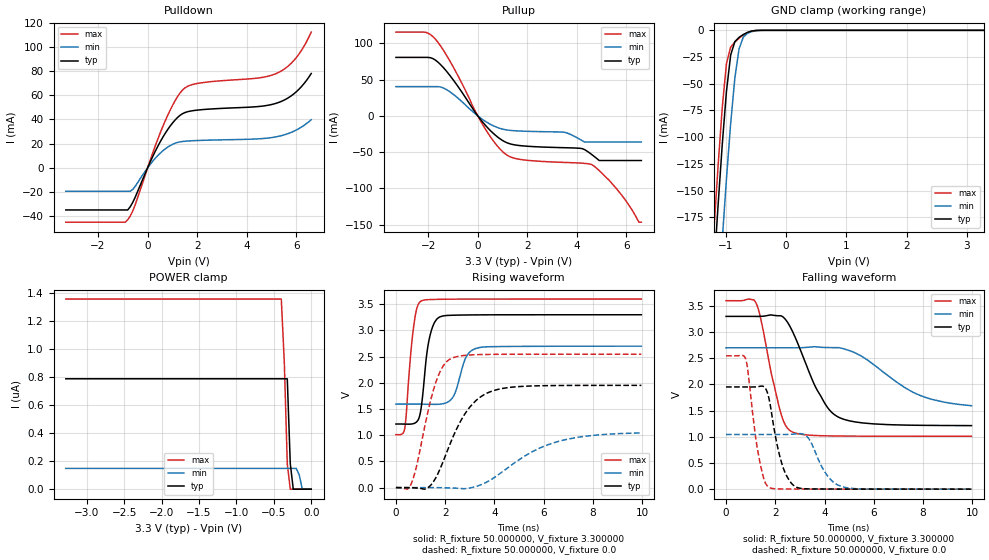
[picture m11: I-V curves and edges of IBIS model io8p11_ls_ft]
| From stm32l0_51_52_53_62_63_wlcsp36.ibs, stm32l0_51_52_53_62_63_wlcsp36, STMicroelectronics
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|   Model io8p11_ls_ft
[Model]  io8p11_ls_ft
Model_type I/O
Polarity   Non-Inverting
Enable   Active-Low
Vinl =   0.990000V
Vinh =   2.310000V
Vmeas =  1.650000V
Cref =   50.000000pF
Rref =   100.000000M
Vref =   0.0V
C_comp   4.606100pF   4.563500pF   4.706200pF
[Temperature Range]   25.000000   0.125000k   -40.000000
[Pullup Reference]   3.300000V   2.700000V   3.600000V
[Pulldown Reference]   0.0V   0.0V   0.0V
[POWER Clamp Reference]   3.300000V   2.700000V   3.600000V
[GND Clamp Reference]   0.0V   0.0V   0.0V
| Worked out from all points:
|   slope of the pulldown table from 0 to 0.495 V, typ, clamps not added: 23.6 ohm
|   slope of the pullup table from 0 to 0.495 V, typ, clamps not added: 24.9 ohm
|   GND clamp passes 1 mA (typ) near -0.59 V on its own axis
|   rising waveform, R_fixture 50.000000, V_fixture 3.300000: 20-80 % time 320ps typ, 429ps min, 283ps max; typ from 1.21 V to 3.3 V
|   rising waveform, R_fixture 50.000000, V_fixture 0.0: 20-80 % time 1.23ns typ, 2.23ns min, 756ps max; typ from 0 V to 1.95 V
|   falling waveform, R_fixture 50.000000, V_fixture 3.300000: 20-80 % time 1.2ns typ, 2.06ns min, 695ps max; typ from 3.3 V to 1.21 V
|   falling waveform, R_fixture 50.000000, V_fixture 0.0: 20-80 % time 523ps typ, 688ps min, 437ps max; typ from 1.95 V to 0 V
[Pulldown]
|Voltage   I(typ)   I(min)   I(max)
-3.3V     -34.78mA   -19.34mA   -44.89mA
-900mV    -34.78mA   -19.34mA   -44.89mA
-800mV    -34.78mA   -19.34mA   -42.84mA
-600mV    -28.56mA   -17.8mA    -35.75mA
100mV     4.638mA    2.744mA    6.076mA
600mV     24.8mA     13.84mA    33.52mA
1V        36.93mA    19.39mA    51.35mA
1.4V      44.67mA    21.76mA    64.17mA
2V        47.71mA    22.58mA    69.7mA
5.2V      53.44mA    25.71mA    78.05mA
6V        62.9mA     31.28mA    91.14mA
6.6V      77.96mA    39.76mA    112.2mA
[Pullup]
|Voltage   I(typ)   I(min)   I(max)
-3.3V     80.5mA     40.22mA    115.4mA
-2.1V     80.5mA     40.22mA    115.1mA
-1.7V     76.61mA    40.22mA    105.3mA
-1.1V     54.57mA    32.56mA    74.14mA
300mV     -12.7mA    -7.45mA    -17.83mA
1.2V      -37.42mA   -19.62mA   -54.57mA
3.5V      -43.95mA   -22.7mA    -64.24mA
4.2V      -45.08mA   -33.97mA   -65.24mA
4.6V      -53.38mA   -36mA      -67.23mA
4.9V      -61.63mA   -36mA      -75.5mA
6.5V      -61.63mA   -36mA      -146.6mA
6.6V      -61.63mA   -36mA      -146.6mA
[GND_clamp]
|Voltage   I(typ)   I(min)   I(max)
-3.3V     -2.275A    -2.356A    -2.249A
-1.2V     -226mA     -318.7mA   -189.2mA
-1.13V    -164.9mA   -256.6mA   -128.3mA
-1.06V    -107.5mA   -196.5mA   -72.78mA
-990mV    -57.32mA   -139.4mA   -31.39mA
-920mV    -23.22mA   -87.32mA   -15.73mA
-850mV    -10.58mA   -44.45mA   -10.94mA
-780mV    -6.539mA   -17.25mA   -7.356mA
-710mV    -3.933mA   -6.349mA   -4.308mA
-640mV    -1.955mA   -2.79mA    -1.975mA
-360mV    -2.06uA    -16.21uA   -459.5nA
3.28V     0A         0A         0A
[POWER_clamp]
|Voltage   I(typ)   I(min)   I(max)
-3.28V    786.7nA    148nA      1.355uA
-400mV    786.7nA    148nA      1.355uA
-360mV    786.7nA    148nA      908.2nA
-320mV    786.7nA    148nA      180.5nA
-280mV    182.6nA    148nA      0A
-240mV    0A         148nA      0A
-200mV    0A         148nA      0A
-160mV    0A         101.6nA    0A
-120mV    0A         0A         0A
0V        0A         0A         0A
[Ramp]
| variable   typ   min   max
dV/dt_r  1.17075/1.22497n   0.60767/2.14101n   1.52754/0.75520n
dV/dt_f  1.24938/1.19094n   0.57786/1.85327n   1.55280/0.69352n
R_load = 50.000000
[Rising Waveform]
R_fixture= 50.000000
V_fixture= 3.300000
V_fixture_min= 2.700000
V_fixture_max= 3.600000
|time   V(typ)   V(min)   V(max)
0s        1.214V     1.593V     1.011V
360.4ps   1.212V     1.593V     1.136V
720.7ps   1.222V     1.593V     3.075V
1.041ns   1.577V     1.593V     3.566V
1.341ns   2.809V     1.59V      3.589V
1.782ns   3.257V     1.592V     3.594V
2.342ns   3.291V     1.747V     3.597V
2.843ns   3.295V     2.484V     3.598V
3.223ns   3.297V     2.653V     3.599V
9.97ns    3.3V       2.7V       3.599V
[Rising Waveform]
R_fixture= 50.000000
V_fixture= 0.0
V_fixture_min= 0.0
V_fixture_max= 0.0
|time   V(typ)   V(min)   V(max)
0s        415.7uV    51.61uV    -108.2uV
620.6ps   -2.248mV   116.2uV    72.4mV
1.221ns   -21.78mV   300.8uV    1.278V
1.582ns   156.7mV    -214.2uV   1.952V
1.882ns   456.7mV    -2.231mV   2.293V
2.202ns   836.7mV    -6.109mV   2.453V
3.003ns   1.538V     -7.5mV     2.531V
4.044ns   1.862V     207.6mV    2.544V
6.547ns   1.948V     874.6mV    2.546V
9.97ns    1.952V     1.044V     2.546V
[Falling Waveform]
R_fixture= 50.000000
V_fixture= 3.300000
V_fixture_min= 2.700000
V_fixture_max= 3.600000
|time   V(typ)   V(min)   V(max)
0s        3.3V       2.7V       3.599V
1.221ns   3.298V     2.7V       3.551V
1.401ns   3.299V     2.7V       3.269V
2.202ns   3.311V     2.7V       1.492V
2.643ns   3.066V     2.699V     1.105V
3.704ns   1.889V     2.716V     1.023V
4.545ns   1.381V     2.702V     1.015V
5.506ns   1.267V     2.539V     1.012V
7.888ns   1.219V     1.788V     1.011V
9.97ns    1.214V     1.593V     1.011V
[Falling Waveform]
R_fixture= 50.000000
V_fixture= 0.0
V_fixture_min= 0.0
V_fixture_max= 0.0
|time   V(typ)   V(min)   V(max)
0s        1.952V     1.044V     2.546V
800.8ps   1.952V     1.044V     2.481V
1.321ns   1.96V      1.044V     645.8mV
1.762ns   1.691V     1.044V     30.75mV
2.282ns   464mV      1.044V     4.004mV
2.863ns   37.01mV    1.056V     2.484mV
3.323ns   5.752mV    986.5mV    1.673mV
4.104ns   2.869mV    265.1mV    795.9uV
4.665ns   2.145mV    56.21mV    467.2uV
9.97ns    415.7uV    51.61uV    -108.2uV
